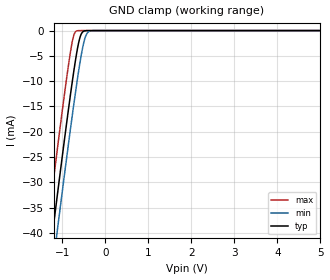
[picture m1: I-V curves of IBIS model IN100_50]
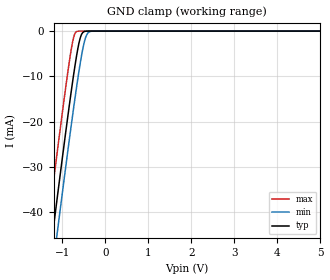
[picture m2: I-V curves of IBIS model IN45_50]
| TEXAS INSTRUMENTS INCORPORATED - Standard Linear and
|   Logic Group / High Volume Linear
| EMI Filter with Integrated VCC Clamp for SIM Card Interface
| Part#   VCC Voltage Range   Package-type   #pins
|TPD3F303DCT   4.5 to 5.5V   SOT   8
[IBIS Ver]   3.2
[Comment char]  |_char
[File Name]   tpd3f303dct.ibs
[File Rev]   1.0 | A0
[Date]   Feburary 24, 2011
[Source]   Data created from TI-SPICE simulations at TI-SLL/HVL.
   The following is an IBIS list for the TPD3F303.
   Please contact sllibis@ti.com with questions and
   comments concerning SLL IBIS models.
[Notes]   Revision History:
   1.0: 02/24/2011
   - Initial version of the model
   - This file contains package information for the SOT 8-pin
   (DCT) package as [Component] TPD3F303_DCT
   - This device can be powered at 5 volt Vcc
[Disclaimer]
| This model is designed as an aid for customers of Texas Instruments.
| TI and its licensors and suppliers make no warranties, either expressed
| or implied, with respect to this  model, including the warranties of
| merchantability or fitness for a particular purpose. The model is
| provided solely on an "as is" basis. The entire risk as to its quality
| and performance is with the customer.
[Copyright]
| (C) Copyright 2011 Texas Instruments Incorporated. All rights reserved.
| Component TPD3F303_DCT 8-PIN SOT
[Component]   TPD3F303_DCT
[Manufacturer]   Texas Instruments, Inc.
[Package]
|   typ   min   max
R_pkg   2.900e-02   2.800e-02   3.100e-02
L_pkg   1.796e-09   1.666e-09   1.924e-09
C_pkg   2.310e-13   2.210e-13   2.420e-13
[Pin]   signal_name   model_name   R_pin   L_pin   C_pin
1   DATA1_Out  IN100_50   3.100e-02   1.894e-09   2.230e-13
2   CLK_OUT   IN45_50   2.800e-02   1.697e-09   2.370e-13
3   DATA2_Out  IN100_50   3.000e-02   1.722e-09   2.390e-13
4   NC   NC   3.000e-02   1.861e-09   2.210e-13
5   VCC   POWER   2.800e-02   1.924e-09   2.280e-13
6   DATA2_In   IN100_50   2.900e-02   1.736e-09   2.420e-13
7   CLK_IN   IN45_50   2.800e-02   1.666e-09   2.360e-13
8   DATA1_In   IN100_50   3.000e-02   1.871e-09   2.220e-13
| Models and submodels in the file (2): IN100_50 (Input), IN45_50 (Input)
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[Model]   IN100_50
Model_type  Input
Vinl=1.75
Vinh=3.25
| variable   typ   min   max
C_comp   17.24pF   12.91pF   23.85pF
[Temperature Range]   40   100   -40
| Ambient temperature   25   85   -40
[Voltage range]   5   4.5   5.5
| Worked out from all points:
|   GND clamp passes 1 mA (typ) near -0.57 V on its own axis
[GND Clamp]
| IN100_50
|   Voltage   I(typ)   I(min)   I(max)
-5V       -304.8mA   -311.4mA   -296.4mA
-1.35V    -48.74mA   -55.7mA    -39.68mA
-1.23V    -40.56mA   -47.53mA   -31.47mA
-1.13V    -33.79mA   -40.77mA   -24.71mA
-1.095V   -31.44mA   -38.42mA   -22.36mA
-800mV    -12.27mA   -19.04mA   -3.895mA
-730mV    -8.099mA   -14.67mA   -974.8uA
-665mV    -4.585mA   -10.76mA   -86.23uA
-580mV    -1.209mA   -6.047mA   -1.421uA
-495mV    -110.6uA   -2.294mA   -21.2nA
-350mV    -579.4nA   -83.81uA   -365.9pA
5V        5.011nA    6.712nA    5.01nA
[Model]   IN45_50
Model_type  Input
Vinl=1.75
Vinh=3.25
| variable   typ   min   max
C_comp   20.30pF   15.19pF   25.90pF
[Temperature Range]   40   100   -40
| Ambient temperature   25   85   -40
[Voltage range]   5   4.5   5.5
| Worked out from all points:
|   GND clamp passes 1 mA (typ) near -0.57 V on its own axis
[GND Clamp]
| IN45_50
|   Voltage   I(typ)   I(min)   I(max)
-5V       -338.2mA   -345.5mA   -328.8mA
-1.35V    -54.14mA   -61.88mA   -44.07mA
-1.23V    -45.07mA   -52.82mA   -34.97mA
-1.13V    -37.56mA   -45.32mA   -27.46mA
-1.095V   -34.95mA   -42.7mA    -24.86mA
-800mV    -13.68mA   -21.21mA   -4.36mA
-730mV    -9.046mA   -16.35mA   -1.094mA
-665mV    -5.137mA   -12.01mA   -90.13uA
-580mV    -1.356mA   -6.772mA   -1.423uA
-495mV    -115.4uA   -2.577mA   -21.2nA
-350mV    -579.6nA   -86.35uA   -365.9pA
5V        5.011nA    6.712nA    5.01nA
